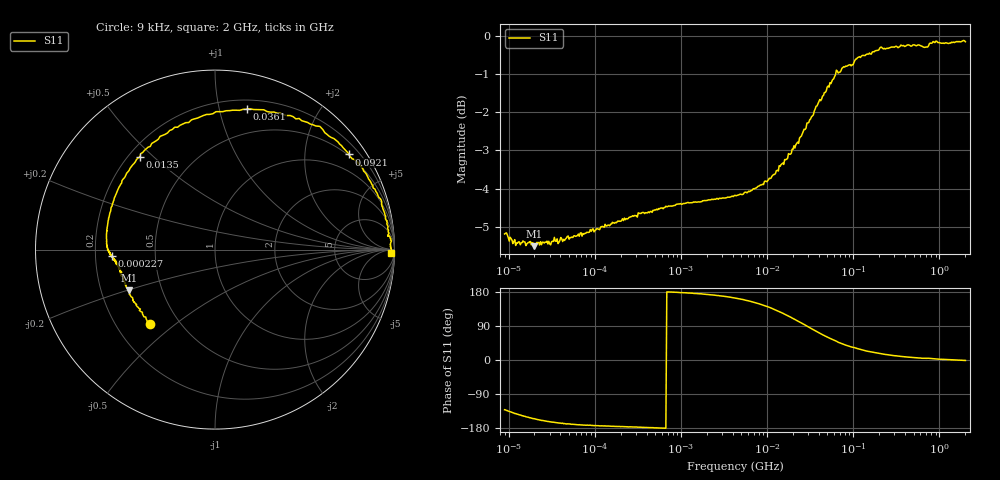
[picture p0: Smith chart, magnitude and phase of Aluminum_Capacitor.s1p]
#  HZ  Z  RI  R  50.0
! 1 port S parameter measurement of a 47 µF aluminum electrolytic capacitor mounted in a 0805 case
! (Panasonic EEEFP1C470AP)
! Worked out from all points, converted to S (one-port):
!   501 points, 9 kHz to 2 GHz, reference 50 ohm
!   lowest |S11| = -5.5 dB at 19.8 kHz (marker M1), VSWR 3.26, Z = 16 - j10.1 ohm
!   |S11| at or under -10 dB: nowhere
!   S11 on the Smith chart (normalised r, x): 9 kHz: 0.34, -0.41; 227 kHz: 0.27, -0.03; 13.5 MHz: 0.24, +0.45; 36.1 MHz: 0.28, +1.21; 92.1 MHz: 0.46, +3.08; 2 GHz: 49, -55
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9000  0.3438 -0.4083
14700  0.3232 -0.267
19800  0.3207 -0.2018
42500  0.3042 -0.1063
74800  0.2916 -0.0648
200000  0.2729 -0.0336
227000  0.2706 -0.0304
922000  0.2483 0.0124
2240000  0.2432 0.0647
4350000  0.2415 0.1401
8250000  0.2394 0.2753
1.06e7  0.2394 0.3541
1.35e7  0.2446 0.4536
1.73e7  0.2475 0.583
2e7  0.2502 0.6758
2.76e7  0.265 0.9254
3.61e7  0.277 1.212
4.86e7  0.3079 1.626
6.53e7  0.3175 2.207
7.75e7  0.3709 2.614
9.21e7  0.4646 3.076
9.44e7  0.5022 3.138
1.33e8  0.6075 4.374
2.08e8  0.814 6.759
2.86e8  1.575 9.417
4.35e8  3 14.45
1e9  24.83 41.35
2e9  49.22 -54.69
